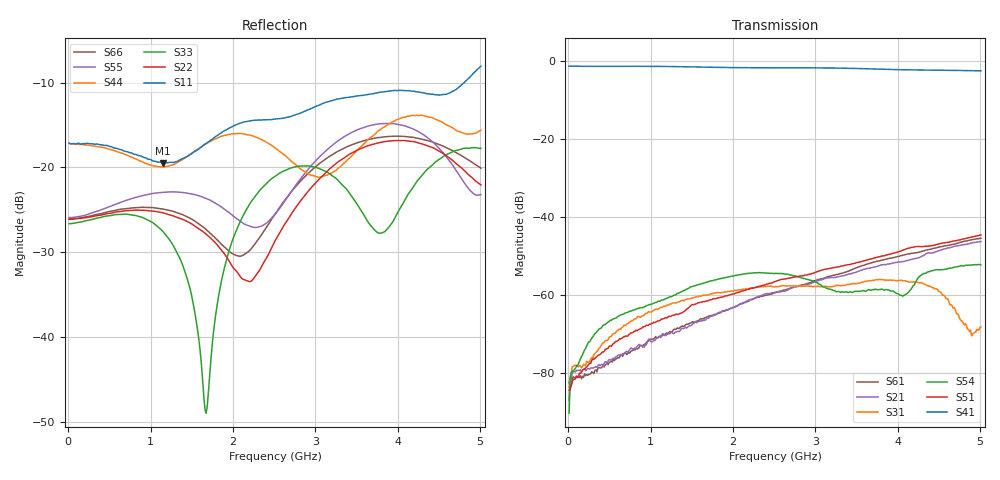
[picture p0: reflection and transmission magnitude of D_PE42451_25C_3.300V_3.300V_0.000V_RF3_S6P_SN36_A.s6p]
! Device ID: PE42451
! Serial: 36
! Insertion: A
! Temp: 25C
! VDD: 3.300
! Control_Hi: 100.000
! Control_Lo: 0.000
! Logic State: RF3
! Port 1: RFC
! Port 2: RF1
! Port 3: RF2
! Port 4: RF3
! Port 5: RF4
! Port 6: RF5
! V1 = 3.30
! V2 = 3.30
! V3 = 0.00
! V4 = 0.00
! IDD: 1.596140e-05
#  Hz  S  RI  R  50
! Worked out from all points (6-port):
!   401 points, 10 MHz to 5.01 GHz, reference 50 ohm
!   strongest paths, dB at 10 MHz, 1.26 GHz, 2.51 GHz, 3.76 GHz, 5.01 GHz:
!     S41: -1.4, -1.5, -1.8, -2.2, -2.6
!     S51: -84.4, -65.3, -56.6, -50.3, -44.7
!     S54: -90.4, -60.4, -54.5, -58.7, -52.3
!     S31: -83.7, -62.1, -57.9, -56.1, -68.2
!     S21: -87.0, -69.7, -59.4, -52.6, -46.4
!     S61: -82.4, -69.6, -59.5, -51.3, -45.5
!   lowest |S11| = -19.5 dB at 1.147 GHz (marker M1), VSWR 1.24, Z = 56.8 - j9.14 ohm
!   |S11| at or under -10 dB: start of sweep to 4.807 GHz
